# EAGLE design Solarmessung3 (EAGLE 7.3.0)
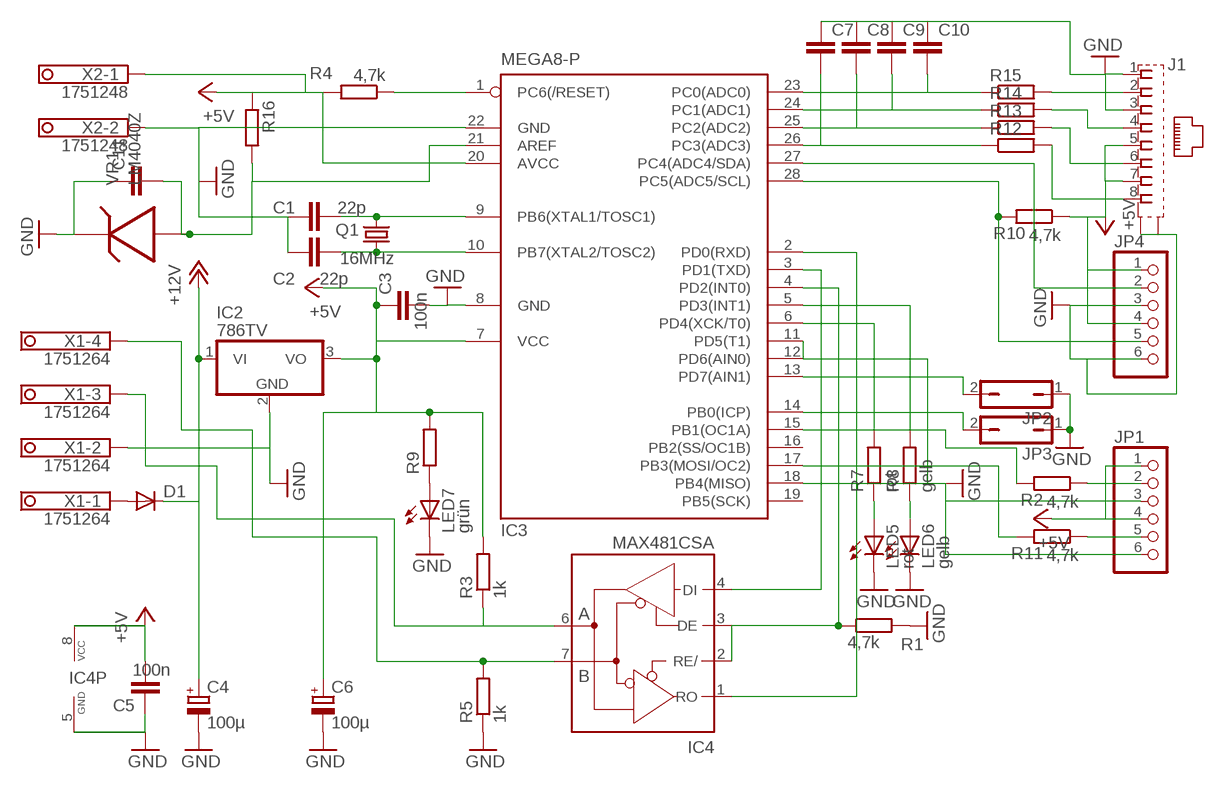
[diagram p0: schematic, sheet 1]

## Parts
C1  22p  C-EUC0603  [C0603]
C2  22p  C-EUC0603  [C0603]
C3  100n  C-EUC0603  [C0603]
C4  100µ  CPOL-EUSMCD  [SMC_D]
C5  100n  C-EU075-032X103  [C075-032X103]
C6  100µ  CPOL-EUSMCD  [SMC_D]
C7  C-EUC0603  [C0603]
C8  C-EUC0603  [C0603]
C9  C-EUC0603  [C0603]
C10  C-EUC0603  [C0603]
C11  C-EUC1206  [C1206]
D1  DIODE-DO214AA  [DO214AA]
IC2  786TV  [TO220V]
IC3  MEGA8-P  [DIL28-3]
IC4  MAX481CSA  [SO08]
J1  557730-1  [557730-1]
JP1  PINHD-1X6  [1X06]
JP2  JP1Q  [JP1]
JP3  JP1Q  [JP1]
JP4  PINHD-1X6  [1X06]
LED5  rot  LED3MM  [LED3MM]
LED6  gelb  LED3MM  [LED3MM]
LED7  grün  LED3MM  [LED3MM]
Q1  16MHz  CRYSTALHC49S  [HC49/S]
R1  4,7k  R-EU_R0603  [R0603]
R2  4,7k  R-EU_R0603  [R0603]
R3  1k  R-EU_R1206  [R1206]
R4  4,7k  R-EU_R0603  [R0603]
R5  1k  R-EU_R1206  [R1206]
R7  rot  R-EU_R0603  [R0603]
R8  gelb  R-EU_R0603  [R0603]
R9  R-EU_R0603  [R0603]
R10  4,7k  R-EU_R0603  [R0603]
R11  4,7k  R-EU_R0603  [R0603]
R12  R-EU_R0603  [R0603]
R13  R-EU_R0603  [R0603]
R14  R-EU_R0603  [R0603]
R15  R-EU_R0603  [R0603]
R16  R-EU_R0603  [R0603]
VR1  LM4040Z  [TO92]
X1  1751264  [1751264]
X2  1751248  [1751248]

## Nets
+5V: C3.1 C5.2 C6.+ IC2.3(VO) IC3.7(VCC) IC3.20(AVCC) IC4.8(VCC) J1.5 J1.7 JP1.1 JP1.4 JP4.1 JP4.4 R3.2 R4.2 R9.2 R10.1 R16.1 X2.1
+12V: C4.+ D1.C IC2.1(VI)
GND: C1.1 C2.1 C3.2 C4.- C5.1 C6.- C7.1 C8.1 C9.1 C10.1 C11.1 IC2.2(GND) IC3.8(GND) IC3.11(PD5(T1)) IC3.12(PD6(AIN0)) IC3.18(PB4(MISO)) IC3.22(GND) IC4.5(GND) J1.1 J1.3 J1.G1(S2) J1.G2(S1) JP1.3 JP1.6 JP2.1 JP3.1 JP4.3 JP4.6 LED5.K(C) LED6.K(C) LED7.K(C) R1.2 R5.1 VR1.1 X1.2 X2.2
N$1: D1.A X1.1
N$2: IC3.2(PD0(RXD)) IC4.1(RO)
N$3: IC4.6(A) R3.1 X1.3
N$4: IC4.7(B) R5.2 X1.4
N$5: IC3.17(PB3(MOSI/OC2)) R11.2
N$6: IC3.13(PD7(AIN1)) JP2.2
N$7: IC3.15(PB1(OC1A)) R2.2
N$8: LED7.A R9.1
N$9: J1.2 R15.2
N$10: IC3.1(PC6(/RESET)) R4.1
N$11: C2.2 IC3.10(PB7(XTAL2/TOSC2)) Q1.1
N$12: C1.2 IC3.9(PB6(XTAL1/TOSC1)) Q1.2
N$13: IC3.3(PD1(TXD)) IC4.4(DI)
N$14: IC3.14(PB0(ICP)) JP3.2
N$15: IC3.4(PD2(INT0)) IC4.2(RE/) IC4.3(DE) R1.1
N$16: C7.2 IC3.26(PC3(ADC3)) R12.1
N$17: J1.6 R13.2
N$18: J1.8 R12.2
N$19: IC3.27(PC4(ADC4/SDA)) JP4.2
N$20: IC3.28(PC5(ADC5/SCL)) JP4.5 R10.2
N$21: JP1.2 R2.1
N$22: JP1.5 R11.1
N$23: C8.2 IC3.25(PC2(ADC2)) R13.1
N$24: C9.2 IC3.24(PC1(ADC1)) R14.1
N$25: C10.2 IC3.23(PC0(ADC0)) R15.1
N$26: J1.4 R14.2
N$27: C11.2 IC3.21(AREF) R16.2 VR1.2
N$36: IC3.6(PD4(XCK/T0)) R7.2
N$37: IC3.5(PD3(INT1)) R8.2
N$38: LED5.A R7.1
N$39: LED6.A R8.1
Unconnected: IC3.16(PB2(SS/OC1B)) IC3.19(PB5(SCK))

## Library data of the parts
C1-C3 C5 C7-C11 = rcl:C-EU: CAPACITOR, European symbol
C4 C6 = rcl:CPOL-EU: POLARIZED CAPACITOR, European symbol
D1 = diode:DIODE-: DIODE
IC2 = linear:78*: Positive VOLTAGE REGULATOR Source: http://cache.national.com/ds/LM/LM78L05.pdf http://www.fairchildsemi.com/ds/LM/LM7805.pdf
IC3 = atmel:MEGA8-P: MICROCONTROLLER 8 Kbytes FLASH, 1 kbytes SRAM, 512 bytes EEPROM, USART, 4-channel 10 bit ADC, 2-channel 8 bit ADC Pin compatible with Atmega48, ATMega88, ATMega168 Source: avr.lbr
IC4 = maxim:MAX481CSA: RS485 TRANSEIVER
J1 = con-amp:557730-1: AMP connector
JP1 JP4 = pinhead:PINHD-1X6: PIN HEADER
JP2 JP3 = jumper:JP1Q: JUMPER
LED5-LED7 = led:LED: LED
Q1 = crystal:CRYSTAL: CRYSTAL
R1-R5 R7-R16 = rcl:R-EU_: RESISTOR, European symbol
VR1 = synthdiy:LM4040: Shunt VOLTAGE REG.
X1 = con-phoenix-350:1751264: MKDS 1/ 4-3,5 Printklemme Nennstrom: 10 A Bemessungsspannung: 160 V Raster: 3,5 mm Polzahl: 4 Montageart: Löten Anschlussart: Schraubanschluss Anschlussrichtung vom Leiter zur Platine: 0° Source: http://eshop.phoenixcontact.com .. 1751264.pdf
X2 = con-phoenix-350:1751248: MKDS 1/ 2-3,5 Printklemme

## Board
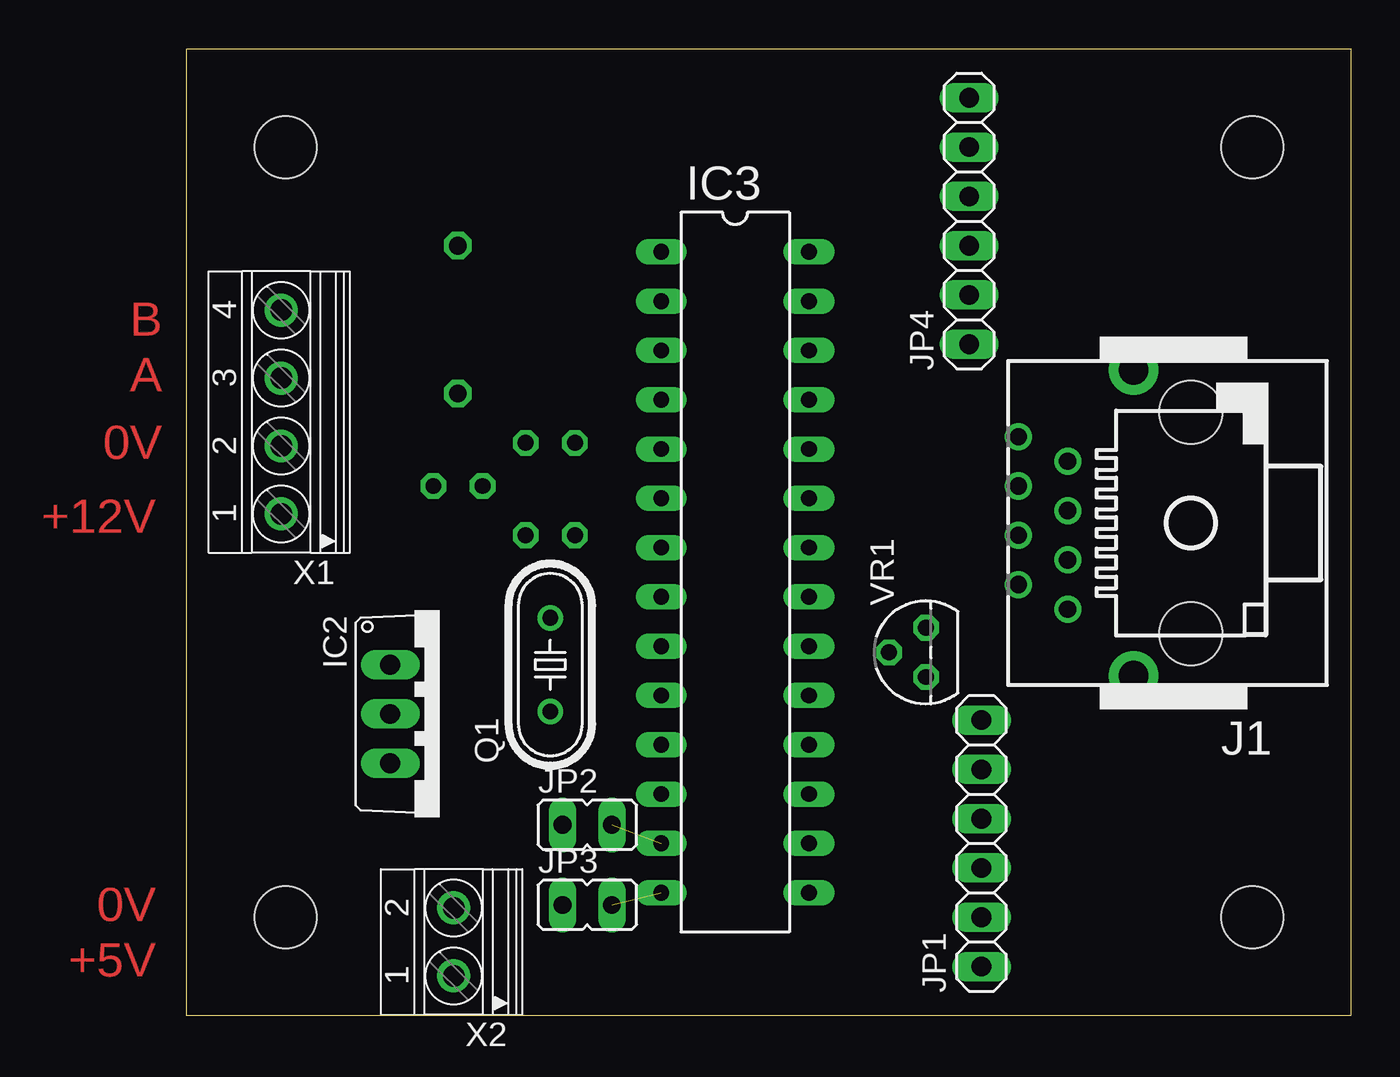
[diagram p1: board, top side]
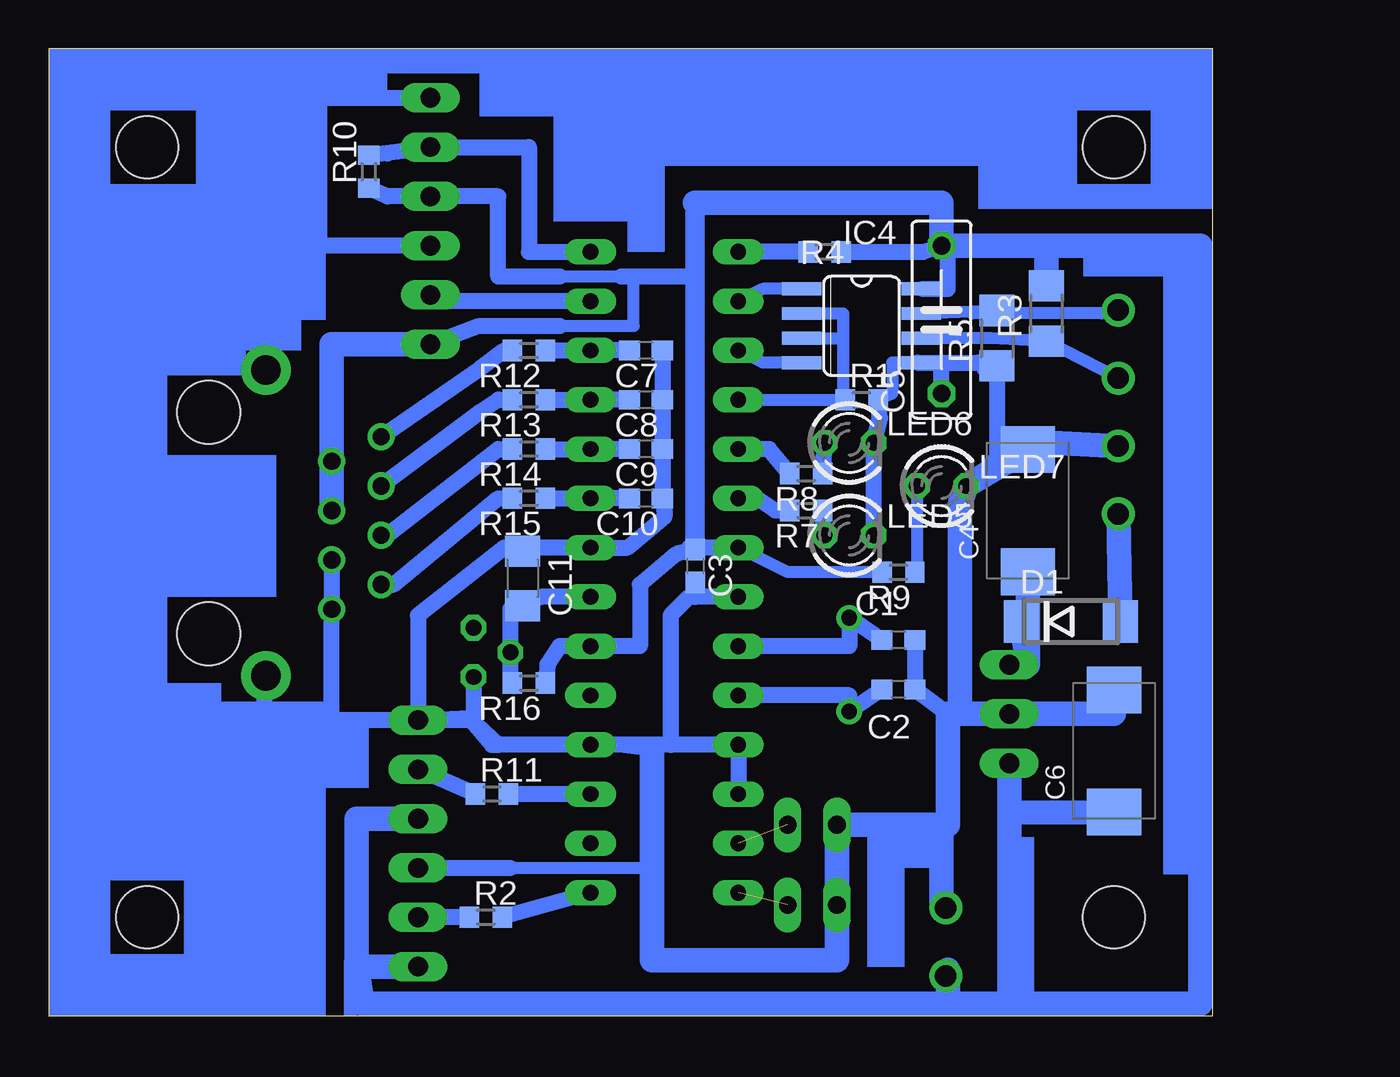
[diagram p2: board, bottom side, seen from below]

Size 60.01 x 49.85 mm. Coordinates in mm from the lower left corner, seen from the top.
Outline: 0,49.85 60.01,49.85 60.01,0 0,0 0,49.85
Copper layers (1*16): Top 0.035mm / dielectric 1.5mm / Bottom 0.035mm
Design rules "default": minimum track width 10mil, minimum drill 24mil, track to track 8mil, track to pad 8mil, pad to pad 8mil, via to via 8mil, smd to smd 8mil, copper to edge 40mil, drill to drill 8mil, minimum pad ring 10mil, minimum via ring 8mil, stop-mask expansion 4mil, vias tented up to drill 0mil, thermal gap 10mil
Holes 3.2 mm at 5.08,44.77 5.08,5.08 54.93,44.77 54.93,5.08

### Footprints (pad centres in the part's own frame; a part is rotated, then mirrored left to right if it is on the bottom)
C0603 = smd 1.1 x 1: 1 -0.85,0; 2 0.85,0
SMC_D = smd 2.4 x 2.8: + -3.15,0; - 3.15,0
C075-032X103 = drill 0.914 octagon: 1 -3.81,0; 2 3.81,0
C1206 = smd 1.6 x 1.8: 1 -1.4,0; 2 1.4,0
DO214AA = smd 1.8 x 2.2: A 2.55,0; C -2.55,0
TO220V = drill 1.016 long: 1 -2.54,-2.54; 2 0,-2.54; 3 2.54,-2.54
DIL28-3 = drill 0.813 long: 1 -16.51,-3.81; 2 -13.97,-3.81; 3 -11.43,-3.81; 4 -8.89,-3.81; 5 -6.35,-3.81; 6 -3.81,-3.81; 7 -1.27,-3.81; 8 1.27,-3.81; 9 3.81,-3.81; 10 6.35,-3.81; 11 8.89,-3.81; 12 11.43,-3.81; 13 13.97,-3.81; 14 16.51,-3.81; 15 16.51,3.81; 16 13.97,3.81; 17 11.43,3.81; 18 8.89,3.81; 19 6.35,3.81; 20 3.81,3.81; 21 1.27,3.81; 22 -1.27,3.81; 23 -3.81,3.81; 24 -6.35,3.81; 25 -8.89,3.81; 26 -11.43,3.81; 27 -13.97,3.81; 28 -16.51,3.81
SO08 = smd 0.66 x 2.032: 1 -1.905,-3.073; 2 -0.635,-3.073; 3 0.635,-3.073; 4 1.905,-3.073; 5 1.905,3.073; 6 0.635,3.073; 7 -0.635,3.073; 8 -1.905,3.073
557730-1 = drill 0.889: 1 -4.445,6.35; 2 -3.175,8.89; 3 -1.905,6.35; 4 -0.635,8.89; 5 0.635,6.35; 6 1.905,8.89; 7 3.175,6.35; 8 4.445,8.89 | drill 1.524 pad 2.54: G1 -7.874,2.946; G2 7.874,2.946 | hole 3.251: -5.715,0; 5.715,0
1X06 = drill 1.016 long: 1 -6.35,0; 2 -3.81,0; 3 -1.27,0; 4 1.27,0; 5 3.81,0; 6 6.35,0
JP1 = drill 0.914 long: 1 0,-1.27; 2 0,1.27
LED3MM = drill 0.813 octagon: A -1.27,0; K 1.27,0
HC49/S = drill 0.813: 1 -2.413,0; 2 2.413,0
R0603 = smd 1 x 1.1: 1 -0.85,0; 2 0.85,0
R1206 = smd 1.6 x 1.803: 1 -1.422,0; 2 1.422,0
TO92 = drill 0.813 octagon: 1 -1.27,0; 2 0,1.905; 3 1.27,0
1751264 = drill 1.1 pad 1.7: 1 -5.25,-0.1; 2 -1.75,-0.1; 3 1.75,-0.1; 4 5.25,-0.1
1751248 = drill 1.1 pad 1.7: 1 -1.75,-0.1; 2 1.75,-0.1

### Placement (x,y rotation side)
C1  16.19,19.37 180 bottom
C2  16.19,16.83 180 bottom
C3  26.67,23.18 270 bottom
C4  9.53,26.04 90 bottom
C5  13.97,35.88 90 bottom
C6  5.08,13.65 90 bottom
C7  29.21,34.29 180 bottom
C8  29.21,31.75 180 bottom
C9  29.21,29.21 180 bottom
C10  29.21,26.67 180 bottom
C11  35.56,22.54 270 bottom
D1  7.3,20.32 0 bottom
IC2  13.02,15.56 270 top
IC3  28.26,22.86 270 top
IC4  18.1,35.56 270 bottom
J1  51.75,25.4 90 top
JP1  40.96,8.89 90 top
JP2  20.64,9.84 270 top
JP3  20.64,5.71 270 top
JP4  40.32,40.96 90 top
LED5  18.73,24.77 0 bottom
LED6  18.73,29.53 0 bottom
LED7  13.97,27.3 0 bottom
Q1  18.73,18.1 90 top
R1  18.1,31.75 0 bottom
R2  37.47,5.08 0 bottom
R3  8.57,36.2 90 bottom
R4  20,39.37 0 bottom
R5  11.11,34.92 90 bottom
R7  20.95,26.04 180 bottom
R8  20.95,27.94 180 bottom
R9  16.19,22.86 180 bottom
R10  43.5,43.5 90 bottom
R11  37.15,11.43 0 bottom
R12  35.24,34.29 180 bottom
R13  35.24,31.75 180 bottom
R14  35.24,29.21 180 bottom
R15  35.24,26.67 180 bottom
R16  35.24,17.14 180 bottom
VR1  38.1,18.73 90 top
X1  4.76,31.11 90 top
X2  13.65,3.81 90 top

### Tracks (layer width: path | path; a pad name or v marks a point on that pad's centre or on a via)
+5V
  Bottom 0.61: R9.2 21.91,22.86 IC3.7 C3.1 | IC4.8 14.92,37.47 | 33.66,38.1 30.48,38.1 | 33.66,35.56 29.84,35.56 29.84,38.1
  Bottom 0.813: IC3.7 26.67,24.13 26.99,24.13 | R10.1 42.55,42.23 JP4.4 36.83,42.23 36.83,38.1 33.66,38.1 | JP4.1 37.78,35.56 33.66,35.56 | C3.1 27.62,23.81 29.53,22.23 29.53,19.05 IC3.20 33.66,19.05 34.29,18.1 R16.1 | 30.48,38.1 29.84,38.1 26.67,38.1 | 14.92,37.47 13.65,37.47 13.65,39.05 C5.2 14.92,39.37 R4.2
  Bottom 1.016: 26.67,24.13 26.67,38.1 26.67,41.91
  Bottom 1.27: IC2.3 10.48,10.48 | 10.48,10.48 C6.+ | JP1.1 44.13,2.54 | 44.13,2.54 44.13,10.16 JP1.4 | 8.57,39.69 0.64,39.69 0.64,0.64 10.48,0.64 | 8.57,39.69 C5.2 13.97,41.91 26.67,41.91 | R3.2 8.57,39.69 | 10.48,0.64 13.65,0.64 | 10.48,10.48 10.48,0.64 | X2.1 13.65,2.38 13.65,0.64 | 13.65,0.64 43.81,0.64 44.13,2.54 | JP4.1 45.4,34.61 J1.7 J1.5
+12V
  Bottom 1.27: D1.C 9.53,18.1 | IC2.1 9.53,18.1 | 9.53,18.1 C4.+
GND
  Bottom 0.406: J1.G2 48.9,33.27
  Bottom 0.61: 36.2,7.62 28.89,7.62 | 28.89,13.65 31.43,13.97 | C3.2 26.67,21.59 | LED7.K 11.11,28.89 | R1.2 16.51,32.07 16.51,33.66 15.24,33.66 IC4.5
  Bottom 0.813: 46.04,39.69 46.04,47.31 JP4.6 | J1.3 J1.1 45.4,15.24 | JP4.3 46.04,39.69 | 46.04,39.69 48.58,39.69 | 48.58,39.69 54.29,39.69 54.29,15.24 48.9,15.24 | 27.94,13.97 IC3.11 IC3.12 | 27.94,13.97 31.43,13.97 IC3.18 36.83,13.97 | 36.83,13.97 37.15,13.97 38.3,15.34 | 36.83,13.97 38.3,15.34 | 38.3,15.34 40.32,15.24 JP1.6 | JP1.6 45.4,15.24 | R5.1 11.11,28.89 C4.- | 11.75,33.34 R5.1 | 13.65,15.56 C2.1 C1.1 | IC3.8 26.67,21.59 26.99,21.59 27.94,20.64 27.94,13.97 | JP1.3 36.2,7.62 | LED5.K LED6.K 17.14,30.8 R1.2 | 48.9,15.24 45.4,15.24 | J1.G1 48.9,17.53 48.9,15.24 | 48.9,33.27 48.9,33.34 48.58,33.34 48.58,39.69 | C7.1 C8.1 C9.1 C10.1 28.26,26.04 28.26,25.72 30.16,24.13 IC3.22 35.88,24.13 | VR1.1 38.1,15.24 JP1.6 | 35.88,24.13 36.51,24.13 40.96,20.64 JP1.6 | C11.1 35.88,24.13 | 15.24,33.66 13.97,33.66 | 13.97,33.66 12.06,33.66 R5.1 | C5.1 13.97,33.66
  Bottom 1.27: X1.2 8.26,29.53 10.79,29.53 C4.- LED7.K 13.02,26.35 13.02,15.56 | 13.02,15.56 IC2.2 5.08,15.56 C6.- | JP3.1 JP2.1 | JP2.1 13.97,9.84 | 13.97,9.84 13.65,9.84 13.65,15.56 13.02,15.56 | JP2.1 19.37,2.86 28.89,2.86 28.89,7.62 28.89,13.65 | X2.2 13.97,5.88 13.97,9.84
N$1
  Bottom 1.27: X1.1 D1.A
N$2
  Bottom 0.61: IC4.1 23.18,37.47 IC3.2
N$3
  Bottom 0.61: X1.3 R3.1 11.43,34.92 IC4.6
N$4
  Bottom 0.61: X1.4 5.71,36.2 12.38,36.2 R5.2 14.29,36.2 IC4.7
N$5
  Bottom 0.813: IC3.17 R11.2
N$6  (1 unrouted)
N$7
  Bottom 0.813: IC3.15 R2.2
N$8
  Bottom 0.61: LED7.A 15.24,22.86 R9.1
N$9
  Bottom 0.813: J1.2 42.23,22.23 36.83,26.67 R15.2
N$10
  Bottom 0.813: R4.1 IC3.1
N$11
  Bottom 0.813: C2.2 Q1.1 18.73,16.51 IC3.10
N$12
  Bottom 0.813: C1.2 Q1.2 18.73,19.05 IC3.9
N$13
  Bottom 0.61: IC4.4 23.18,33.66 IC3.3
N$14  (1 unrouted)
N$15
  Bottom 0.61: IC4.2 19.05,36.2 19.05,34.92 | IC3.4 R1.1 19.05,32.07 19.05,34.92 | IC4.3 19.05,34.92
N$16
  Bottom 0.813: C7.2 IC3.26 R12.1
N$17
  Bottom 0.813: J1.6 37.78,31.11 36.83,31.75 R13.2
N$18
  Bottom 0.813: J1.8 37.78,33.34 36.51,34.29 R12.2
N$19
  Bottom 0.813: IC3.27 39.37,36.83 JP4.2
N$20
  Bottom 0.813: R10.2 42.55,44.45 JP4.5 35.24,44.77 35.24,39.37 IC3.28
N$21
  Bottom 0.813: R2.1 JP1.2
N$22
  Bottom 0.813: R11.1 JP1.5
N$23
  Bottom 0.813: C8.2 IC3.25 R13.1
N$24
  Bottom 0.813: C9.2 IC3.24 R14.1
N$25
  Bottom 0.813: C10.2 IC3.23 R15.1
N$26
  Bottom 0.813: J1.4 42.55,24.77 36.83,29.21 R14.2
N$27
  Bottom 0.813: R16.2 36.2,17.04 VR1.2 36.2,20.95 C11.2 34.61,21.59 IC3.21
N$36
  Bottom 0.813: R7.2 22.54,26.04 23.5,26.67 IC3.6
N$37
  Bottom 0.813: R8.2 22.86,29.21 IC3.5
N$38
  Bottom 0.813: LED5.A R7.1
N$39
  Bottom 0.813: LED6.A R8.1
(copper drawn outside any net)
  shapes: Bottom area x48

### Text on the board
Top: B | A | 0V | +12V | 0V | +5V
